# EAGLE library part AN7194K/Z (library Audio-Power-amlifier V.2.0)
The AN7194K and AN7194Z are single power supply, BTL, audio class-H power amplifier ICs. A class-H power amplifier can be made up when this ICs are used in combination with the AN7077Z which is separately market- available, and it is possible to make a low consumption power system. Also, the AN7194K and AN7194Z are incorporating various protection circuits, so that those ICs contribute to the high reliability design of set.
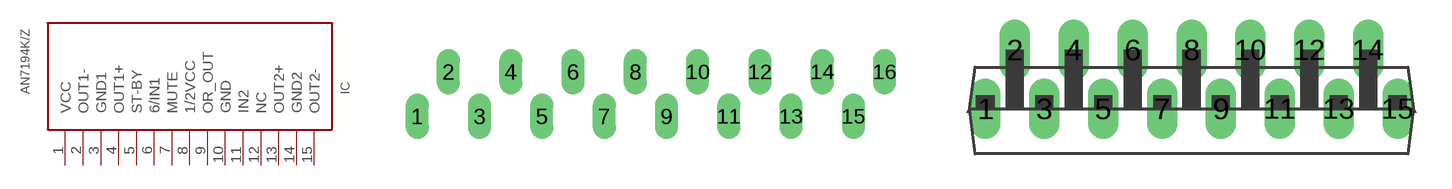
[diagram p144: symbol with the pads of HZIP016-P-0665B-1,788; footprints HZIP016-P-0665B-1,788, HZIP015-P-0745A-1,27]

Designator prefix IC

## AN7194K/ZAN7194K  [HZIP016-P-0665B-1,788]
1  VCC  pwr
2  OUT1-  out
3  GND1  pwr
4  OUT1+  out
5  ST-BY  in
6  6/IN1  in
7  MUTE  in
8  1/2VCC  pwr
9  OR_OUT  out
10  GND  pwr
11  IN2  in
12  NC  nc
13  OUT2+  out
14  GND2  pwr
15  OUT2-  out

## AN7194K/ZAN7194Z  [HZIP015-P-0745A-1,27]
Pads as for HZIP016-P-0665B-1,788

## Footprint HZIP016-P-0665B-1,788 (pad centres in mm)
drill 0.8 long: 1 -13.334,0; 2 -11.556,2.539; 3 -9.778,-0.001; 4 -8,2.539; 5 -6.222,-0.001; 6 -4.444,2.539; 7 -2.666,0; 8 -0.888,2.539; 9 0.889,-0.001; 10 2.668,2.538; 11 4.446,0; 12 6.224,2.539; 13 8,-0.001; 14 9.78,2.539; 15 11.557,-0.001; 16 13.337,2.539

## Footprint HZIP015-P-0745A-1,27 (pad centres in mm)
drill 0.8 long: 1 -8.89,-1.27; 2 -7.62,1.27; 3 -6.35,-1.27; 4 -5.08,1.27; 5 -3.81,-1.27; 6 -2.54,1.27; 7 -1.27,-1.27; 8 0,1.27; 9 1.27,-1.27; 10 2.54,1.27; 11 3.81,-1.27; 12 5.08,1.27; 13 6.35,-1.27; 14 7.62,1.27; 15 8.89,-1.27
